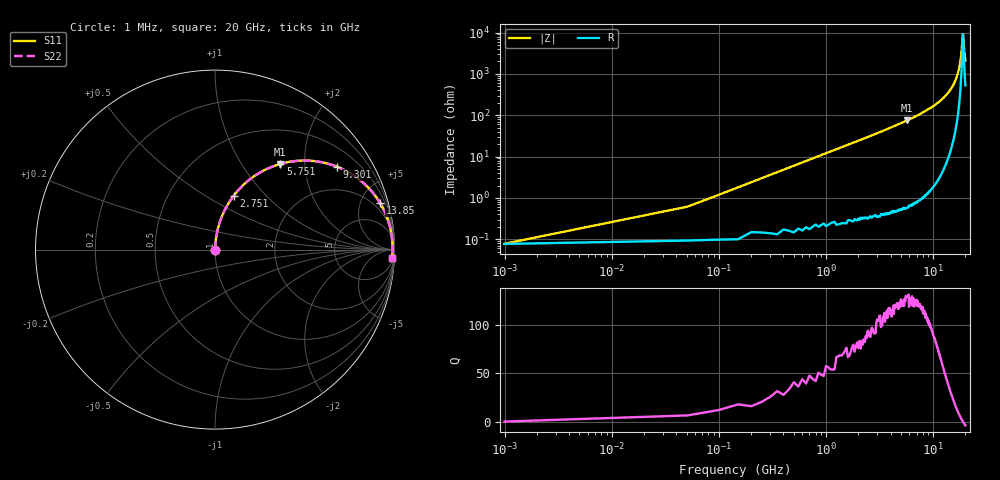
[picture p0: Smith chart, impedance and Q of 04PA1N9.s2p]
! Coilcraft 0402PA-1N9 Chip Inductor
! 11 March 2004
# MHZ S MA R 50
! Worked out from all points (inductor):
!   401 points, 1 MHz to 20 GHz, reference 50 ohm
!   read as one part in series: L = 1.9 nH near 101 MHz
!   highest Q = 130 at 5.701 GHz (marker M1), where L = 2.09 nH
!   self-resonance near 18.95 GHz
!   S11 on the Smith chart (normalised r, x): 1 MHz: 1.00, +0.00; 2.751 GHz: 1.01, +0.67; 5.751 GHz: 1.01, +1.51; 9.301 GHz: 1.03, +2.92; 13.85 GHz: 1.18, +7.07; 20 GHz: 12, -41
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1  0.0005575 12.3  0.999 -0.0  0.999 -0.0  0.0005575 12.3
150.993  0.018 85.3  0.999 -1.0  0.999 -1.0  0.018 85.3
300.985  0.036 85.6  0.998 -2.1  0.998 -2.1  0.036 85.6
500.975  0.06 84.9  0.997 -3.4  0.997 -3.4  0.06 84.9
850.957  0.101 83.0  0.993 -5.8  0.993 -5.8  0.101 83.0
1300.935  0.154 80.2  0.986 -8.8  0.986 -8.8  0.154 80.2
2750.862  0.317 70.9  0.945 -18.5  0.945 -18.5  0.317 70.9
3350.832  0.38 67.1  0.921 -22.4  0.921 -22.4  0.38 67.1
5700.715  0.597 52.9  0.798 -36.6  0.798 -36.6  0.597 52.9
5750.713  0.601 52.6  0.795 -36.9  0.795 -36.9  0.601 52.6
6700.665  0.672 47.3  0.735 -42.2  0.735 -42.2  0.672 47.3
9300.535  0.821 34.2  0.562 -55.2  0.562 -55.2  0.821 34.2
10000.5  0.851 31.0  0.515 -58.4  0.515 -58.4  0.851 31.0
13350.33  0.947 17.5  0.3 -71.2  0.3 -71.2  0.947 17.5
13850.31  0.956 15.7  0.27 -72.8  0.27 -72.8  0.956 15.7
16700.17  0.985 6.4  0.112 -79.0  0.112 -79.0  0.985 6.4
18050.1  0.989 2.5  0.045 -74.6  0.045 -74.6  0.989 2.5
18400.08  0.989 1.6  0.029 -67.8  0.029 -67.8  0.989 1.6
18950.05  0.989 0.1  0.011 -8.7  0.011 -8.7  0.989 0.1
19150.04  0.989 -0.4  0.013 33.9  0.013 33.9  0.989 -0.4
19600.02  0.988 -1.6  0.03 66.1  0.03 66.1  0.988 -1.6
20000  0.987 -2.6  0.047 72.9  0.047 72.9  0.987 -2.6
